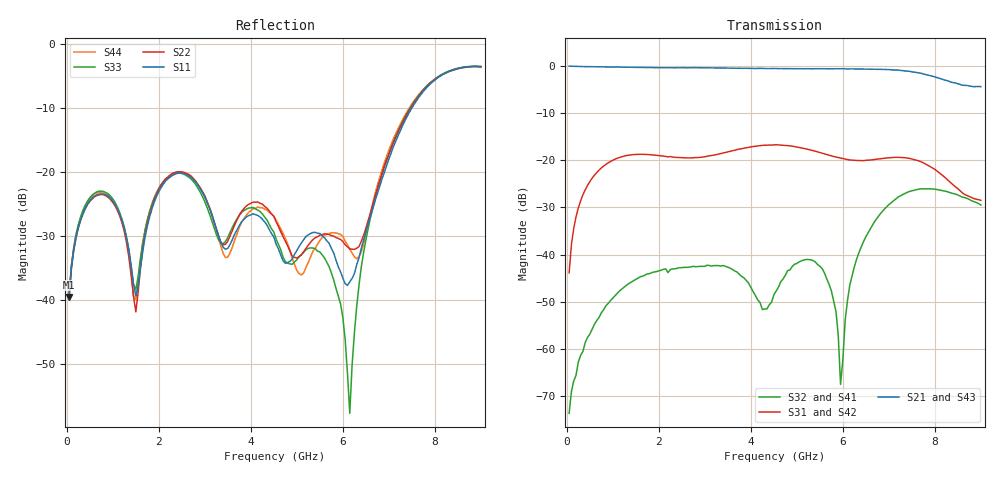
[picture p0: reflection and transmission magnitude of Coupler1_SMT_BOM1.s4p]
! Created Tue Sep 05 15:50:36 2017
# hz S ma R 50
! 4 Port Network Data from SP1.SP block
! freq  magS11  angS11  magS12  angS12  magS13  angS13  magS14  angS14
!  magS21  angS21  magS22  angS22  magS23  angS23  magS24  angS24
!  magS31  angS31  magS32  angS32  magS33  angS33  magS34  angS34
!  magS41  angS41  magS42  angS42  magS43  angS43  magS44  angS44
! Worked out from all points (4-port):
!   180 points, 50 MHz to 9 GHz, reference 50 ohm
!   strongest paths, dB at 50 MHz, 2.3 GHz, 4.55 GHz, 6.8 GHz, 9 GHz:
!     S21: -0.1, -0.4, -0.5, -0.7, -4.4
!     S43: -0.1, -0.4, -0.5, -0.7, -4.5
!     S31: -43.9, -19.3, -16.7, -19.7, -28.5
!     S42: -43.9, -19.3, -16.7, -19.7, -28.5
!     S32: -73.6, -43.0, -47.7, -31.5, -29.5
!     S41: -73.6, -43.0, -47.7, -31.5, -29.5
!   lowest |S11| = -39.5 dB at 50 MHz (marker M1), VSWR 1.02, Z = 50.6 + j0.868 ohm
!   |S11| at or under -10 dB: start of sweep to 7.5 GHz
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5e7  0.01054 54.4  0.9947 -5.5  0.006423 82.6  0.0002242 -135.1
     0.9937 -5.6  0.01054 54.5  0.0002242 -135.1  0.006423 82.6
     0.006403 83.4  0.0002083 -121.5  0.01092 55.7  0.994 -5.5
     0.0002083 -121.5  0.006403 83.4  0.9937 -5.5  0.01088 55.3
1.7e9  0.03093 79.6  0.963 -179.4  0.1154 -89.0  0.006088 -167.0
       0.9607 -179.5  0.0321 70.6  0.006088 -167.0  0.1154 -89.0
       0.1156 -88.9  0.006086 -167.7  0.0348 80.1  0.9623 -179.3
       0.006087 -167.8  0.1156 -88.9  0.9608 -179.4  0.03513 74.5
3.3e9  0.0317 -80.3  0.9504 11.9  0.1162 102.3  0.007772 -44.6
       0.9501 11.8  0.03144 -82.3  0.00777 -44.6  0.1162 102.3
       0.1164 102.4  0.007646 -45.1  0.02947 -65.7  0.9512 12.1
       0.007645 -45.1  0.1164 102.4  0.9492 12.1  0.03069 -98.9
4.3e9  0.04076 -100.8  0.9385 -94.4  0.1445 -4.0  0.002654 -137.6
       0.9385 -94.3  0.05384 -105.5  0.002653 -137.7  0.1446 -4.0
       0.1443 -4.1  0.002654 -139.1  0.04449 -105.8  0.9387 -94.1
       0.002653 -139.2  0.1443 -4.1  0.939 -94.0  0.05131 -112.3
6.15e9  0.01387 -25.0  0.9281 66.1  0.1011 156.7  0.00453 163.2
        0.9302 66.1  0.02511 -100.6  0.004529 163.2  0.1011 156.7
        0.1008 156.7  0.00472 166.3  0.0013 -68.9  0.9287 66.5
        0.004719 166.3  0.1008 156.7  0.9299 66.4  0.02491 -126.1
7.45e9  0.2948 -177.4  0.8748 -82.0  0.105 2.7  0.04666 -56.4
        0.8764 -82.0  0.306 -178.7  0.04666 -56.4  0.105 2.7
        0.1048 2.6  0.04676 -56.4  0.3125 -176.5  0.8691 -81.7
        0.04676 -56.4  0.1048 2.6  0.8719 -81.6  0.3189 -178.2
9e9  0.6664 29.7  0.6021 118.7  0.03757 -96.0  0.03376 72.2
     0.6029 118.8  0.6633 34.7  0.03375 72.2  0.03756 -96.0
     0.03762 -95.4  0.03363 72.9  0.669 34.2  0.5988 119.1
     0.03365 72.9  0.03761 -95.4  0.5974 119.0  0.6642 30.5
